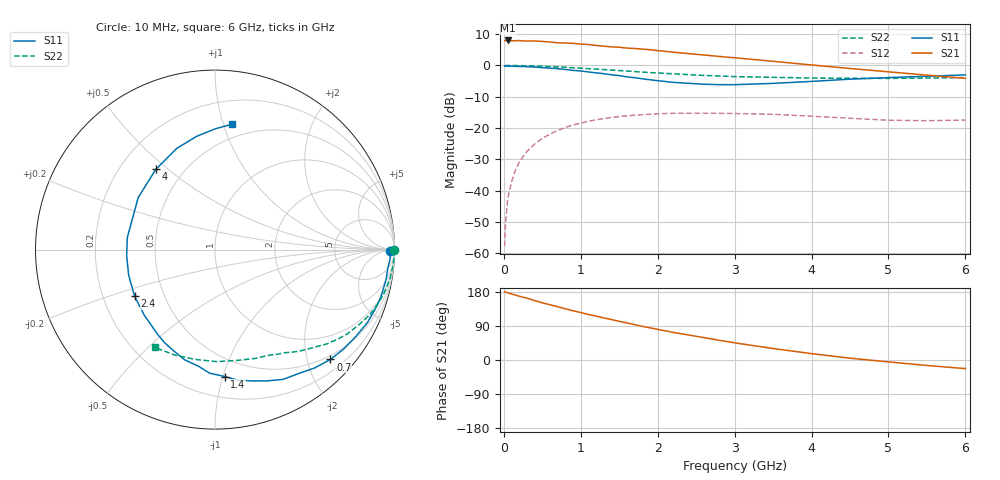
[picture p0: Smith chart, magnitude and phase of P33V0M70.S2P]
! SIEMENS Small Signal Semiconductors
! BFP181
! Si NPN RF Bipolar Junction Transistor in SOT143
! VCE = 3 V  IC = 0.7 mA
! Common Emitter S-Parameters:  March  1996
# GHz  S  MA  R  50
!  f  S11  S21  S12  S22
! GHz  MAG  ANG  MAG  ANG  MAG  ANG  MAG  ANG
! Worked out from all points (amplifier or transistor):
!   36 points, 10 MHz to 6 GHz, reference 50 ohm
!   highest |S21| = 8.0 dB at 50 MHz (marker M1)
!   |S21| within 3 dB of that: start of sweep to 1.914 GHz
!   unconditionally stable (mu >= 1): 3.542 GHz to end of sweep
!   at 250 MHz: K = 0.08, MSG = 18.5 dB, |S12| = -29.1 dB
!   at 1.4 GHz: K = 0.45, MSG = 11.3 dB, |S12| = -16.6 dB
!   at 6 GHz: K = 1.37, MAG = 3.0 dB, |S12| = -17.4 dB
!   S11 on the Smith chart (normalised r, x): 10 MHz: 67, -28; 700 MHz: 0.42, -2.44; 1.4 GHz: 0.36, -1.01; 2.4 GHz: 0.34, -0.24; 4 GHz: 0.35, +0.46; 6 GHz: 0.38, +1.07
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0.01  0.9749 -0.6  2.5 179.8  0.0013 90.4  0.9988 -0.2
0.02  0.9772 -1.3  2.482 179.5  0.0027 86.7  0.9927 -0.6
0.05  0.9774 -2.9  2.506 177.1  0.0075 88.3  0.9977 -1.5
0.1  0.9678 -6.4  2.478 174.4  0.0137 83.1  0.9987 -3.0
0.15  0.9681 -9.6  2.473 171.4  0.0213 82.7  0.9955 -4.5
0.25  0.9608 -15.8  2.463 165.6  0.035 79.1  0.9909 -7.5
0.4  0.9418 -25.5  2.462 156.8  0.0556 72.9  0.9806 -11.9
0.5  0.9217 -31.8  2.417 150.9  0.0683 68.2  0.9719 -14.8
0.7  0.8877 -43.6  2.298 140.6  0.0917 60.4  0.9482 -20.3
0.9  0.8334 -55.9  2.249 129.9  0.112 52.4  0.919 -25.3
1.1  0.7872 -68.3  2.158 120.1  0.1285 45.2  0.8881 -30.0
1.4  0.7093 -85.6  1.977 106.7  0.1475 35.5  0.8434 -36.6
1.5  0.689 -92.5  1.955 102.0  0.1526 32.8  0.8276 -38.3
1.8  0.6113 -111.6  1.825 88.8  0.1635 25.3  0.7836 -43.5
2.2  0.5375 -137.1  1.628 73.0  0.1721 15.6  0.7361 -50.2
2.4  0.518 -149.8  1.546 66.0  0.173 11.4  0.7133 -53.3
3  0.4932 172.2  1.325 45.3  0.1706 1.2  0.6633 -62.2
3.5  0.517 145.8  1.164 30.3  0.1659 -4.8  0.646 -69.9
4  0.5562 126.2  1.018 16.8  0.1546 -9.0  0.6292 -79.1
4.5  0.603 110.7  0.894 4.8  0.1434 -11.4  0.6239 -89.4
5.5  0.673 89.9  0.7 -14.5  0.131 -7.3  0.6288 -110.6
6  0.7059 82.1  0.622 -22.7  0.1344 -4.5  0.6399 -121.6
